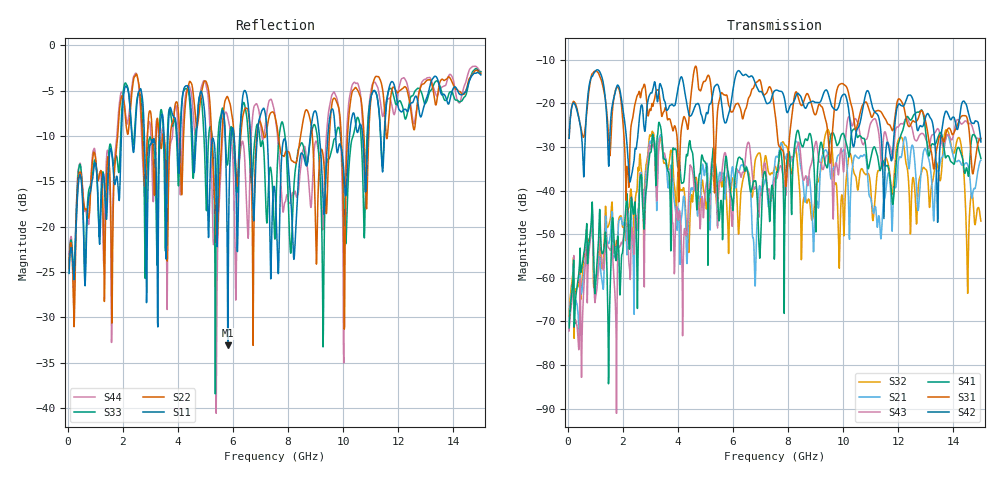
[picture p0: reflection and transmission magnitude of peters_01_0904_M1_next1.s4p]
# MHZ S RI R 50.00
! FREQ  S11  S12  S13  S14
!  S21  S22  S23  S24
!  S31  S32  S33  S34
!  S41  S42  S43  S44
!  REAL  IMAG  REAL  IMAG  REAL  IMAG  REAL  IMAG
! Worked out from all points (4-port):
!   1496 points, 50 MHz to 15 GHz, reference 50 ohm
!   strongest paths, dB at 50 MHz, 3.79 GHz, 7.53 GHz, 11.27 GHz, 15 GHz:
!     S42: -28.0, -20.2, -17.1, -22.9, -28.9
!     S31: -28.1, -25.6, -22.5, -21.6, -28.0
!     S41: -71.5, -33.3, -42.8, -32.8, -32.7
!     S43: -72.2, -45.9, -37.0, -26.0, -28.3
!     S21: -70.5, -35.7, -33.0, -46.7, -33.1
!     S32: -68.8, -31.3, -34.5, -35.4, -47.0
!   lowest |S11| = -33.1 dB at 5.81 GHz (marker M1), VSWR 1.05, Z = 51.6 + j1.58 ohm
!   |S11| at or under -10 dB: start of sweep to 1.947 GHz; 2.782 GHz to 3.344 GHz (561.4 MHz wide, 18.3 % of centre); 7.244 GHz to 8.802 GHz (1.558 GHz wide, 19.4 % of centre)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
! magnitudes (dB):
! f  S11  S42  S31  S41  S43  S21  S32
! 50 MHz  -25.1  -28.0  -28.1  -71.5  -72.2  -70.5  -68.8
! 3.05 GHz  -10.5  -17.7  -20.2  -29.5  -29.7  -28.3  -26.8
! 4.18 GHz  -5.4  -14.9  -24.0  -38.2  -65.8  -42.8  -39.7
! 5.81 GHz  -33.1  -23.0  -19.2  -35.5  -36.5  -35.5  -47.6
! 6.78 GHz  -17.5  -14.9  -15.9  -37.9  -39.7  -57.7  -34.5
! 13.76 GHz  -6.1  -21.9  -26.4  -32.1  -27.5  -27.3  -26.1
! 15 GHz  -3.3  -28.9  -28.0  -32.7  -28.3  -33.1  -47.0
